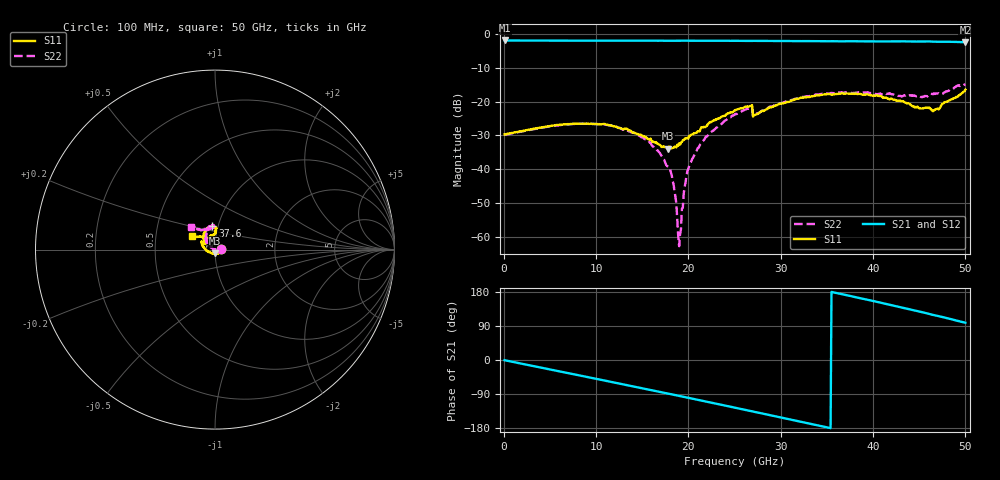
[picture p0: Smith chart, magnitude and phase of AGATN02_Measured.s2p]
! Filename4Jim: AG16_W2_AGATN02_A_0715_LRM_1BW_LRM.s2p
! Calibration: AG02 LRM + TRL
! Notes:
! Row:7, Col:15
! Probes: nan
! Prober: MPI TS150
! Date: 2023-09-21 11:11:43
! DC: None
# GHz S dB R 50
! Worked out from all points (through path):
!   500 points, 100 MHz to 50 GHz, reference 50 ohm
!   highest |S21| = -1.92 dB at 100 MHz (marker M1); lowest = -2.4 dB at 50 GHz (marker M2)
!   group delay of S21, straight-line fit = 14.4 ps
!   lowest |S11| = -33.9 dB at 17.8 GHz (marker M3), VSWR 1.04, Z = 50.1 - j2.02 ohm
!   |S11| at or under -10 dB: start of sweep to end of sweep
!   |S22| runs from -62.7 to -14.9 dB; largest |S21 - S12| = 0.001
!   S11 on the Smith chart (normalised r, x): 100 MHz: 1.07, +0.00; 37.6 GHz: 0.94, +0.25; 50 GHz: 0.76, +0.12
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0.1  -29.71 1.3  -1.92 -0.5  -1.92 -0.5  -29.84 1.3
8.5  -26.53 8.7  -1.98 -42.2  -1.98 -42.2  -26.52 14.7
13.3  -28.01 -16.6  -1.99 -66.0  -1.99 -66.1  -28.41 2.5
15.5  -30.85 -43.5  -1.99 -77.1  -1.99 -77.1  -31.43 -3.8
16.8  -32.68 -66.4  -1.99 -83.7  -1.99 -83.7  -34.88 -6.9
17.8  -33.91 -87.0  -2.00 -88.7  -2.00 -88.7  -39.17 -2.8
18.1  -33.59 -99.8  -1.99 -90.2  -1.99 -90.2  -40.87 -12.7
18.4  -33.63 -105.8  -1.99 -91.7  -1.99 -91.7  -44.47 -17.3
19  -32.33 -119.0  -1.99 -94.8  -1.99 -94.8  -62.75 122.3
19.2  -32.08 -122.8  -1.99 -95.8  -1.99 -95.8  -57.67 128.6
19.5  -31.36 -131.6  -1.98 -97.3  -1.99 -97.3  -47.10 175.3
19.7  -30.82 -138.4  -1.98 -98.3  -1.98 -98.3  -43.81 169.5
20.3  -29.82 -150.9  -1.98 -101.4  -1.98 -101.4  -37.77 159.1
22  -27.16 -170.4  -2.01 -110.2  -2.01 -110.2  -30.34 147.7
25.1  -22.46 161.4  -2.01 -126.1  -2.01 -126.1  -23.60 136.6
26.7  -21.27 149.2  -2.04 -134.4  -2.05 -134.4  -21.84 130.3
27.2  -23.91 148.4  -2.03 -137.1  -2.03 -137.1  -23.78 132.9
33.4  -18.44 115.1  -2.12 -169.4  -2.12 -169.4  -18.20 108.8
37.6  -17.65 96.5  -2.14 168.7  -2.14 168.6  -17.41 95.5
41.7  -19.24 86.5  -2.20 146.4  -2.21 146.4  -17.64 95.7
46.6  -22.57 119.4  -2.28 118.5  -2.28 118.5  -17.59 117.4
50  -16.46 149.8  -2.44 98.3  -2.44 98.3  -14.85 136.8
